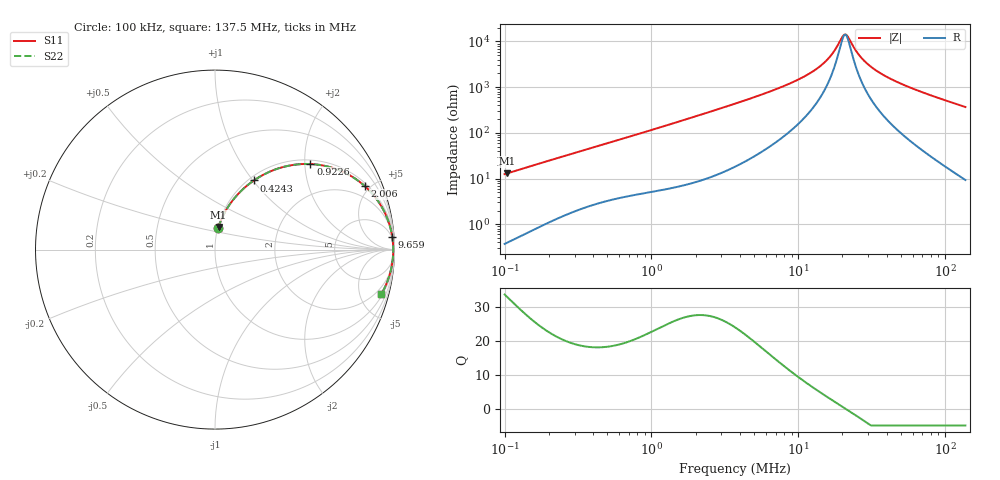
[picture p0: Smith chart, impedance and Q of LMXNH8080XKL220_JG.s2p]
! LMXNH8080XKL220_JG  S-PARAMETER MODEL  ( General Type )
! Model Generated by TAIYO YUDEN Corporation (http://www.ty-top.com)
! Version 1.0
! TAIYO YUDEN Control No. 191025NI43SB-FBB
! Copyright(c) 2019 TAIYO YUDEN CO.,LTD. All Rights Reserved.
! Product Description (link to TY-COMPAS)
! https://ds.yuden.co.jp/TYCOMPAS/or/detail?pn=LMXNH8080XKL220MJG&u=M
! Products Name : Inductors
! Characteristics :
!  Inductance : 22 uH , SRF(min) : 16 MHz , DC Resistance(max) : 0.091 Ohm
!  Rated Current : Saturation :1750 mA , Temp Rise : 1900 mA
!  Case Size : 8.0 x 8.0 / 0.315 x 0.315 [mm/inch] , Thickness : 3 / 0.118 [mm/inch]
!  (Conditions: Temperature = 25 degC , DC Bias Current/Voltage = 0A / 0V)
! External Node Assignments :
!  1  o---GGG---o  2
! GND o---------o GND
! Frequency Range : 0.1MHz  -  137.487582MHz  [ 402 STEP ]
# MHz S RI R 50
! Freq[MHz].  S11 Real  S11 Imag  S21 Real  S21 Imag  S12 Real  S12 Imag  S22 Real  S22 Imag
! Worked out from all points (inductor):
!   401 points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, 100 kHz to 137.5 MHz, reference 50 ohm
!   read as one part in series: L = 19.8 uH near 103.7 kHz
!   highest Q = 33 at 103.7 kHz (marker M1), where L = 19.9 uH
!   self-resonance near 20.63 MHz
!   S11 on the Smith chart (normalised r, x): 100 kHz: 1.01, +0.25; 424.3 kHz: 1.06, +1.01; 922.6 kHz: 1.10, +2.13; 2.006 MHz: 1.17, +4.61; 9.659 MHz: 4, +28; 137.5 MHz: 1.19, -7.36
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0.1  0.0189 0.1221  0.9811 -0.1221  0.9811 -0.1221  0.0189 0.1221
0.103679  0.0202 0.1263  0.9798 -0.1263  0.9798 -0.1263  0.0202 0.1263
0.198671  0.0655 0.2262  0.9345 -0.2262  0.9345 -0.2262  0.0655 0.2262
0.335474  0.1539 0.3348  0.8461 -0.3348  0.8461 -0.3348  0.1539 0.3348
0.42428  0.2166 0.3852  0.7834 -0.3852  0.7834 -0.3852  0.2166 0.3852
0.922605  0.5312 0.4767  0.4688 -0.4767  0.4688 -0.4767  0.5312 0.4767
1.125429  0.6222 0.4642  0.3778 -0.4642  0.3778 -0.4642  0.6222 0.4642
2.006224  0.8332 0.3551  0.1668 -0.3551  0.1668 -0.3551  0.8332 0.3551
3.707932  0.9418 0.2142  0.0582 -0.2142  0.0582 -0.2142  0.9418 0.2142
9.659433  0.9877 0.0702  0.0123 -0.0702  0.0123 -0.0702  0.9877 0.0702
12.43915  0.9909 0.0449  0.00914 -0.0449  0.00914 -0.0449  0.9909 0.0449
16.0188  0.9925 0.0222  0.00751 -0.0222  0.00751 -0.0222  0.9925 0.0222
17.53309  0.9928 0.0146  0.0072 -0.0146  0.0072 -0.0146  0.9928 0.0146
19.89656  0.993 0.00397  0.00698 -0.00397  0.00698 -0.00397  0.993 0.00397
21.00463  0.993 -0.000544  0.00695 0.000544  0.00695 0.000544  0.993 -0.000544
21.77741  0.993 -0.00355  0.00696 0.00355  0.00696 0.00355  0.993 -0.00355
25.62225  0.9928 -0.0172  0.00722 0.0172  0.00722 0.0172  0.9928 -0.0172
28.55559  0.9924 -0.0265  0.00762 0.0265  0.00762 0.0265  0.9924 -0.0265
33.59712  0.9914 -0.0411  0.0086 0.0411  0.0086 0.0411  0.9914 -0.0411
41.73016  0.9892 -0.0622  0.0108 0.0622  0.0108 0.0622  0.9892 -0.0622
69.20356  0.9775 -0.1235  0.0225 0.1235  0.0225 0.1235  0.9775 -0.1235
137.4876  0.9258 -0.2498  0.0742 0.2498  0.0742 0.2498  0.9258 -0.2498
